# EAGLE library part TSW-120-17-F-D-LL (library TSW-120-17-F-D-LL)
CONN HEADER 40 POS .100" Source: Datasheet
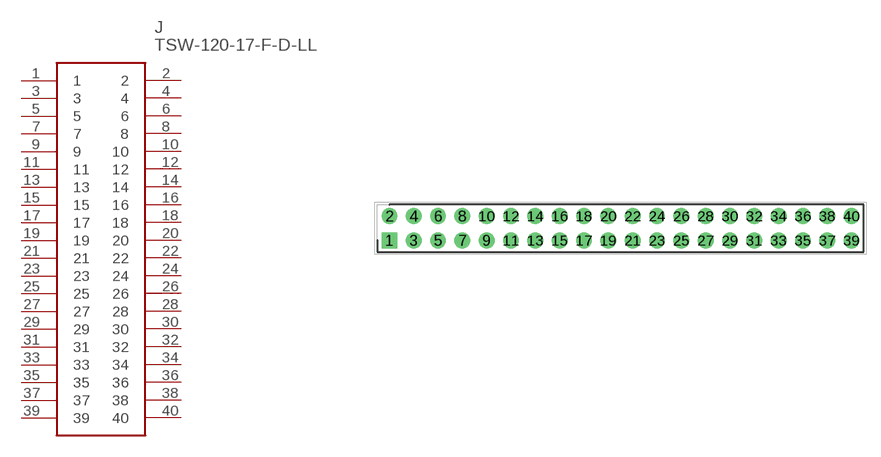
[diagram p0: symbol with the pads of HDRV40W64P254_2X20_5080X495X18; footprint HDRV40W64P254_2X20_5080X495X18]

Designator prefix J

## TSW-120-17-F-D-LL (Description: CONN HEADER 40 POS .100"; Height: 18.28mm; Manufacturer_Name: SAMTEC; Manufacturer_Part_Number: TSW-120-17-F-D-LL)  [HDRV40W64P254_2X20_5080X495X18]
1  1
2  2
3  3
4  4
5  5
6  6
7  7
8  8
9  9
10  10
11  11
12  12
13  13
14  14
15  15
16  16
17  17
18  18
19  19
20  20
21  21
22  22
23  23
24  24
25  25
26  26
27  27
28  28
29  29
30  30
31  31
32  32
33  33
34  34
35  35
36  36
37  37
38  38
39  39
40  40

## Footprint HDRV40W64P254_2X20_5080X495X18 (pad centres in mm)
TSW-120-17-F-D-LL
drill 1.1 pad 1.65 square: 1 0,0
drill 1.1 pad 1.65: 2 0,2.54; 3 2.54,0; 4 2.54,2.54; 5 5.08,0; 6 5.08,2.54; 7 7.62,0; 8 7.62,2.54; 9 10.16,0; 10 10.16,2.54; 11 12.7,0; 12 12.7,2.54; 13 15.24,0; 14 15.24,2.54; 15 17.78,0; 16 17.78,2.54; 17 20.32,0; 18 20.32,2.54; 19 22.86,0; 20 22.86,2.54; 21 25.4,0; 22 25.4,2.54; 23 27.94,0; 24 27.94,2.54; 25 30.48,0; 26 30.48,2.54; 27 33.02,0; 28 33.02,2.54; 29 35.56,0; 30 35.56,2.54; 31 38.1,0; 32 38.1,2.54; 33 40.64,0; 34 40.64,2.54; 35 43.18,0; 36 43.18,2.54; 37 45.72,0; 38 45.72,2.54; 39 48.26,0; 40 48.26,2.54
